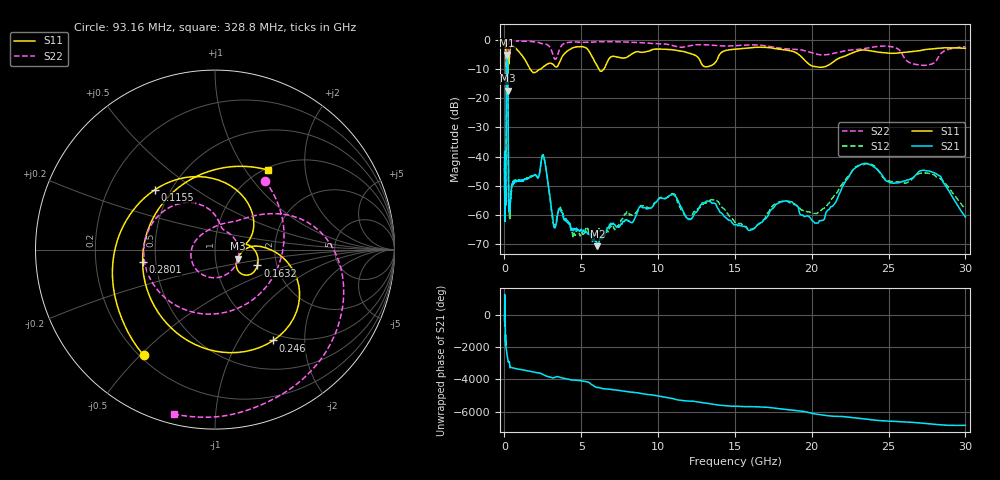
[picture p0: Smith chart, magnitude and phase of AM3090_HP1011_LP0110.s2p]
! Date/Time: Thu, Feb 28, 2019 2:05 PM
! Network Analyzer: Agilent Technologies E8364B Rev: A.07.50.67
! Sweep from 0.010 to 30.000 GHz, 1601 Points, Sweep Type: LOG
! Power Supply: 5.022 V, 0.002 A
# Hz S DB R 50
!freq MagS11 AngS11 MagS21 AngS21 MagS12 AngS12 MagS22 AngS22
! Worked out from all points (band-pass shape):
!   1601 points, 10 MHz to 30 GHz, reference 50 ohm
!   highest |S21| = -5.18 dB at 166.5 MHz (marker M1); lowest = -70.7 dB at 6.049 GHz (marker M2)
!   |S21| within 3 dB of the highest: 130.7 MHz to 214.4 MHz (83.68 MHz wide, 48.5 % of centre)
!   lowest |S11| = -17.4 dB at 198.3 MHz (marker M3), VSWR 1.31, Z = 64 - j6.58 ohm
!   |S11| at or under -10 dB: 125.2 MHz to 220.7 MHz (95.5 MHz wide, 55.2 % of centre); 1.669 GHz to 2.361 GHz (691.6 MHz wide, 34.3 % of centre); 6.144 GHz to 6.469 GHz (325.1 MHz wide, 5.16 % of centre)
!   |S22| runs from -19.0 to -0.2 dB; largest |S21 - S12| = 0.019
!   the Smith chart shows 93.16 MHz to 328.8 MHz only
!   S11 on the Smith chart (normalised r, x): 93.16 MHz: 0.22, -0.51; 115.5 MHz: 0.41, +0.35; 163.2 MHz: 1.58, -0.30; 246 MHz: 0.90, -1.42; 280.1 MHz: 0.42, -0.07; 328.8 MHz: 1.03, +1.28
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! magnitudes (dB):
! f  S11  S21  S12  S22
! 10 MHz  -0.2  -38.2  -43.9  -0.5
! 38.04 MHz  -0.4  -60.6  -58.7  -1.3
! 93.16 MHz  -3.0  -54.5  -52.6  -6.5
! 115.5 MHz  -6.5  -21.9  -21.9  -8.1
! 144.7 MHz  -14.9  -5.8  -5.7  -18.4
! 163.2 MHz  -12.0  -5.2  -5.2  -16.6
! 166.5 MHz  -12.0  -5.2  -5.2  -16.3
! 198.3 MHz  -17.4  -6.0  -6.0  -19.0
! 223.6 MHz  -9.1  -11.8  -11.9  -11.6
! 246 MHz  -4.4  -37.8  -37.8  -2.8
! 280.1 MHz  -7.8  -58.5  -56.0  -1.0
! 328.8 MHz  -5.5  -56.4  -59.3  -0.5
! 550.5 MHz  -2.0  -49.0  -48.8  -0.3
! 2.084 GHz  -10.9  -46.6  -46.6  -0.7
! 2.533 GHz  -9.2  -39.6  -39.5  -1.3
! 3.236 GHz  -8.8  -64.4  -64.6  -6.3
! 6.049 GHz  -9.0  -70.7  -65.8  -0.7
! 7.926 GHz  -6.0  -61.6  -59.4  -0.7
! 10.76 GHz  -3.3  -53.3  -53.2  -1.7
! 20.1 GHz  -9.0  -62.2  -59.5  -4.5
! 23.48 GHz  -3.5  -42.3  -42.5  -2.9
! 30 GHz  -2.9  -60.7  -58.0  -2.3
